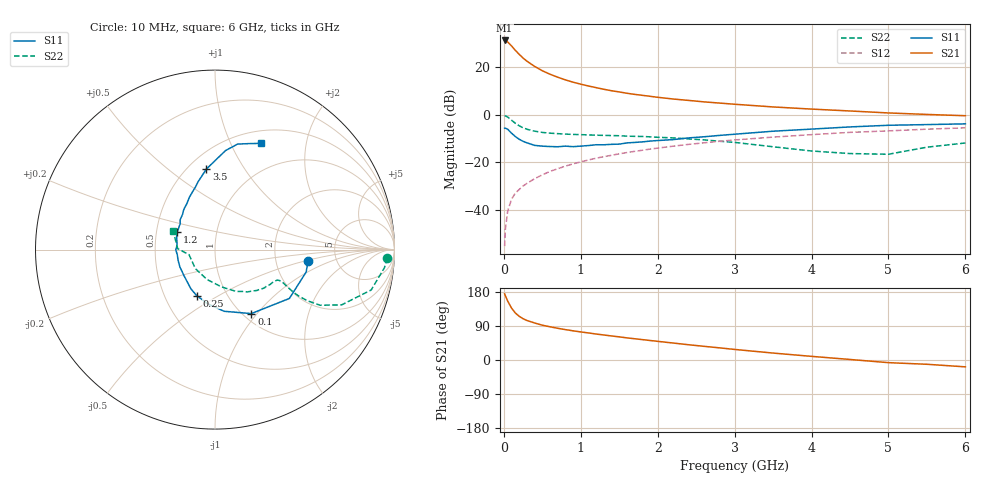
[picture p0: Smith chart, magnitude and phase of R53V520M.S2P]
! SIEMENS Small Signal Semiconductors
! BFR183
! Si NPN RF Bipolar Junction Transistor in SOT23
! VCE = 3.5 V  IC = 20 mA
! Common Emitter S-Parameters:  May  1996
# GHz  S  MA  R  50
!  f  S11  S21  S12  S22
! GHz  MAG  ANG  MAG  ANG  MAG  ANG  MAG  ANG
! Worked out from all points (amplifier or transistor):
!   36 points, 10 MHz to 6 GHz, reference 50 ohm
!   highest |S21| = 31.3 dB at 10 MHz (marker M1)
!   |S21| within 3 dB of that: start of sweep to 118.6 MHz
!   unconditionally stable (mu >= 1): 561 MHz to 2.359 GHz
!   at 250 MHz: K = 0.81, MSG = 27.0 dB, |S12| = -30.0 dB
!   at 1.4 GHz: K = 1.05, MAG = 12.3 dB, |S12| = -17.1 dB
!   at 6 GHz: K = 0.90, MSG = 2.6 dB, |S12| = -5.5 dB
!   S11 on the Smith chart (normalised r, x): 10 MHz: 3.08, -0.54; 100 MHz: 1.09, -0.93; 250 MHz: 0.72, -0.40; 1.2 GHz: 0.64, +0.13; 3.5 GHz: 0.61, +0.69; 6 GHz: 0.65, +1.31
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0.01  0.5221 -7.0  36.92 174.6  0.0017 94.1  0.962 -2.8
0.02  0.5231 -13.8  36.51 169.4  0.0039 81.3  0.9494 -6.1
0.05  0.4958 -33.3  34.24 155.5  0.0093 77.7  0.8988 -14.5
0.1  0.41 -60.4  28.33 137.0  0.0166 72.0  0.7695 -23.6
0.15  0.3474 -81.6  22.81 123.9  0.0224 68.7  0.6626 -27.9
0.2  0.3049 -97.4  18.78 115.3  0.0267 68.6  0.5862 -29.0
0.25  0.2761 -111.6  15.73 108.9  0.0315 68.8  0.5314 -29.0
0.3  0.2565 -121.6  13.5 104.3  0.0358 69.3  0.4962 -28.5
0.4  0.2265 -139.0  10.48 97.7  0.045 70.5  0.4521 -27.2
0.5  0.2183 -153.6  8.489 91.9  0.0542 71.3  0.4255 -26.1
0.6  0.2142 -163.6  7.168 87.6  0.0641 71.5  0.4105 -25.6
0.7  0.212 -172.3  6.206 83.7  0.0729 71.4  0.4003 -25.6
0.8  0.2185 -179.8  5.449 80.2  0.0828 70.7  0.3919 -25.8
0.9  0.2129 173.9  4.869 77.0  0.0924 70.6  0.3856 -26.2
1.1  0.2249 161.9  4.047 71.4  0.1116 69.6  0.3768 -28.1
1.2  0.2337 155.1  3.735 68.5  0.1215 68.9  0.3717 -28.9
1.6  0.2554 139.6  2.847 58.4  0.16 65.1  0.355 -34.2
2.2  0.2998 121.6  2.153 44.8  0.2179 58.7  0.3257 -44.4
3.5  0.4511 96.1  1.465 18.3  0.3384 42.5  0.2117 -79.8
4.5  0.555 83.9  1.204 1.4  0.4262 29.8  0.1523 -136.0
5.5  0.6218 71.8  1.018 -11.3  0.4978 18.1  0.2076 178.6
6  0.6441 66.7  0.956 -18.1  0.5312 10.5  0.2547 156.2
